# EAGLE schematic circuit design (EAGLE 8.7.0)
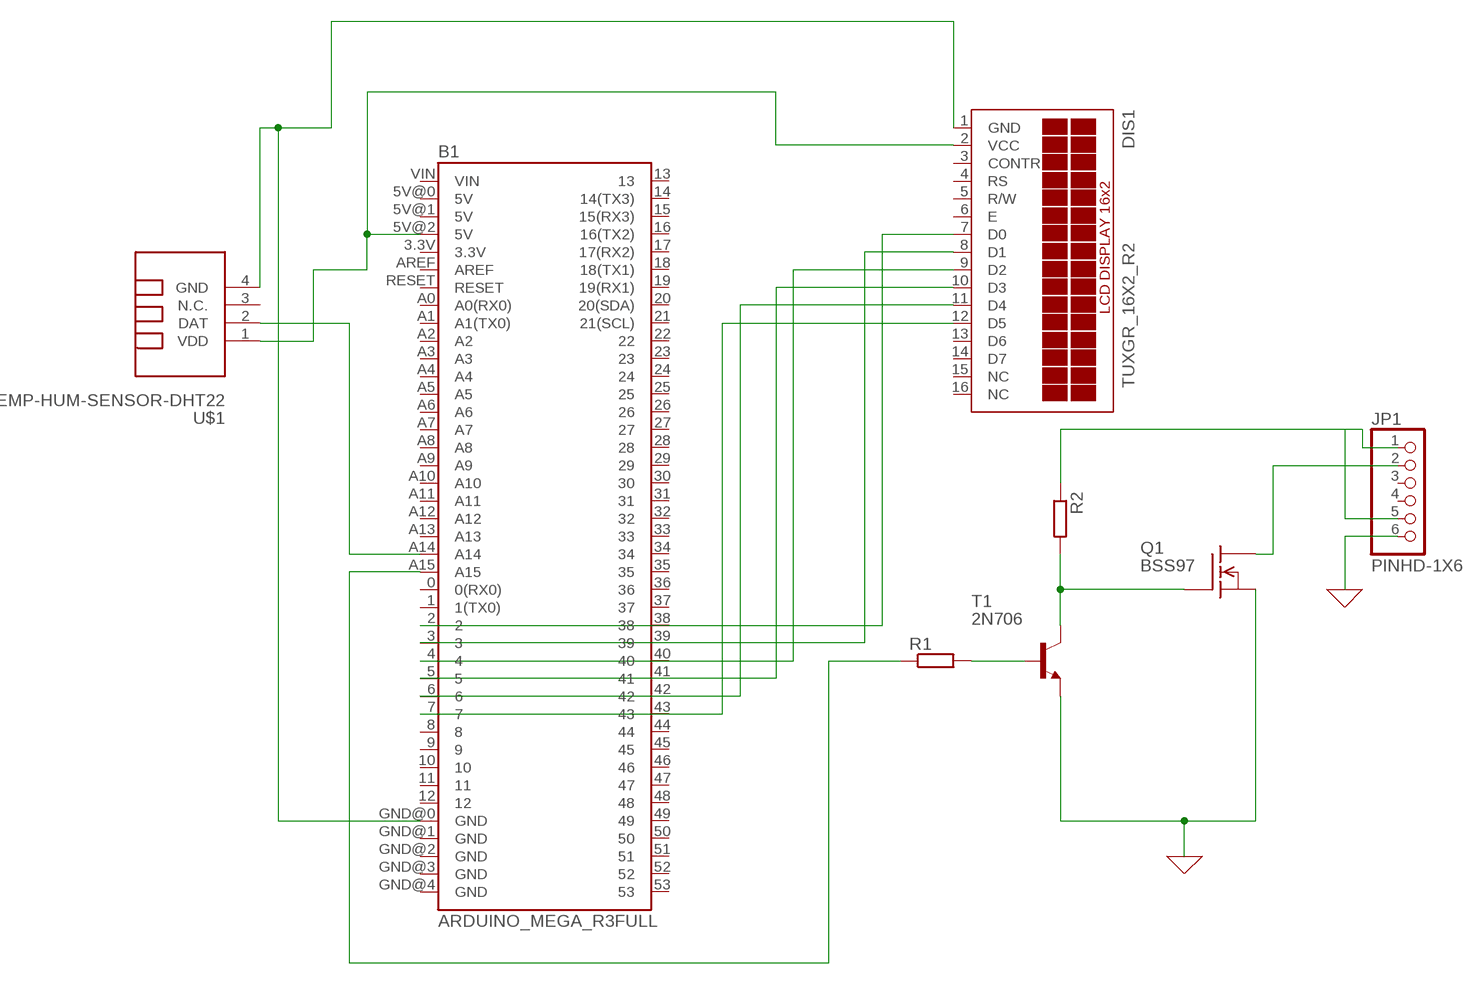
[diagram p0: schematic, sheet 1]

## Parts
B1  ARDUINO_MEGA_R3FULL  [ARDUINO_MEGA]
DIS1  TUXGR_16X2_R2  [TUXGR_16X2_R2]
JP1  PINHD-1X6  [1X06]
Q1  BSS97  [TO202]
R1  R0207/10  [0207/10]
R2  R0207/10  [0207/10]
T1  2N706  [TO18]
U$1  TEMP-HUM-SENSOR-DHT22  [TEMP-HUM-SENSOR-DHT22]

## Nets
0: JP1.6 Q1.1(S) T1.1(E) ; supply symbol labelled GND
N$1: R1.2 T1.2(B)
N$2: Q1.3(G) R2.2 T1.3(C)
N$3: B1.4 DIS1.9(D2)
N$4: JP1.1 JP1.5 R2.1
N$5: JP1.2 Q1.2(D)
N$6: B1.5 DIS1.10(D3)
N$7: B1.A15 R1.1
N$8: B1.A14 U$1.2(DAT)
N$9: B1.5V@2(5V) DIS1.2(VCC) U$1.1(VDD)
N$10: B1.GND@0(GND) DIS1.1(GND) U$1.4(GND)
N$11: B1.2 DIS1.7(D0)
N$12: B1.3 DIS1.8(D1)
N$13: B1.6 DIS1.11(D4)
N$14: B1.7 DIS1.12(D5)
Unconnected: B1.0(0(RX0)) B1.1(1(TX0)) B1.3.3V B1.5V@0(5V) B1.5V@1(5V) B1.8 B1.9 B1.10 B1.11 B1.12 B1.13 B1.14(14(TX3)) B1.15(15(RX3)) B1.16(16(TX2)) B1.17(17(RX2)) B1.18(18(TX1)) B1.19(19(RX1)) B1.20(20(SDA)) B1.21(21(SCL)) B1.22 B1.23 B1.24 B1.25 B1.26 B1.27 B1.28 B1.29 B1.30 B1.31 B1.32 B1.33 B1.34 B1.35 B1.36 B1.37 B1.38 B1.39 B1.40 B1.41 B1.42 B1.43 B1.44 B1.45 B1.46 B1.47 B1.48 B1.49 B1.50 B1.51 B1.52 B1.53 B1.A0(A0(RX0)) B1.A1(A1(TX0)) B1.A2 B1.A3 B1.A4 B1.A5 B1.A6 B1.A7 B1.A8 B1.A9 B1.A10 B1.A11 B1.A12 B1.A13 B1.AREF B1.GND@1(GND) B1.GND@2(GND) B1.GND@3(GND) B1.GND@4(GND) B1.RESET B1.VIN DIS1.3(CONTR) DIS1.4(RS) DIS1.5(R/W) DIS1.6(E) DIS1.13(D6) DIS1.14(D7) DIS1.15(NC) DIS1.16(NC) JP1.3 JP1.4 U$1.3(N.C.)

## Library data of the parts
B1 = SparkFun-Boards:ARDUINO_MEGA_R3: Arduino Mega R3 ATmega2560 R3 compatible footprint. SparkFun Products: Arduino Mega 2560 R3
DIS1 = display-lcd:TUXGR_16X2_R2: Tuxgraphics LCD display 16x2 characters reflective, without background light Source: tuxgr_12x2_r2.pdf; OC_FARNELL: unknown; OC_NEWARK: unknown
JP1 = audio amplifier example:PINHD-1X6: PIN HEADER
Q1 = transistor-fet:BSS97: N-Channel Enhancement MOSFET 200V; 1.5A; 1,6Ohm
R1 R2 = eagle-ltspice:R: RESISTOR, European symbol; SPICEMODEL: NONE; SPICEPREFIX: R
T1 = transistor:2N706: NPN TRANSISTOR
U$1 = diy-modules:TEMP-HUM-SENSOR-DHT22: DHT22 - digital humidity & temperature sensor Also known as: AM2302 AM2302 datasheet available here: http://akizukidenshi.com/download/ds/aosong/AM2302.pdf Click here to find device on ebay.com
